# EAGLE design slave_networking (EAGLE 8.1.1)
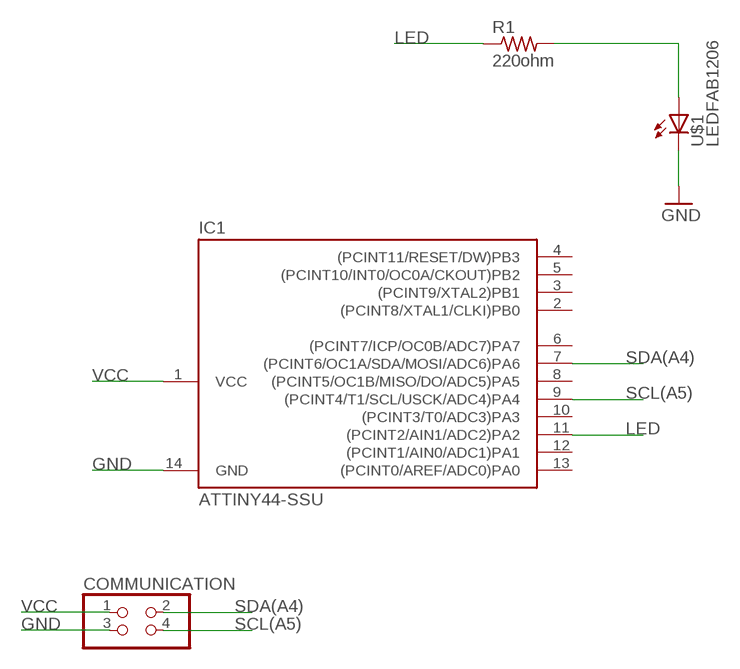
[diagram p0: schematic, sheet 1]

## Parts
COMMUNICATION  PINHD-2X2-SMD  [2X02SMD]
IC1  ATTINY44-SSU  [SOIC14]
R1  220ohm  RES-US1206FAB  [R1206FAB]
U$1  LEDFAB1206  [LED1206FAB]

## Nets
GND: COMMUNICATION.3 IC1.14(GND) U$1.2(C)
LED: IC1.11((PCINT2/AIN1/ADC2)PA2) R1.1
N$1: R1.2 U$1.1(A)
SCL(A5): COMMUNICATION.4 IC1.9((PCINT4/T1/SCL/USCK/ADC4)PA4)
SDA(A4): COMMUNICATION.2 IC1.7((PCINT6/OC1A/SDA/MOSI/ADC6)PA6)
VCC: COMMUNICATION.1 IC1.1(VCC)
Unconnected: IC1.2((PCINT8/XTAL1/CLKI)PB0) IC1.3((PCINT9/XTAL2)PB1) IC1.4((PCINT11/RESET/DW)PB3) IC1.5((PCINT10/INT0/OC0A/CKOUT)PB2) IC1.6((PCINT7/ICP/OC0B/ADC7)PA7) IC1.8((PCINT5/OC1B/MISO/DO/ADC5)PA5) IC1.10((PCINT3/T0/ADC3)PA3) IC1.12((PCINT1/AIN0/ADC1)PA1) IC1.13((PCINT0/AREF/ADC0)PA0)

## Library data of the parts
COMMUNICATION = fab:PINHD-2X2-SMD
IC1 = fab:ATTINY44
R1 = fab:RES-US: Resistor (US Symbol)
U$1 = fab:LED: LED

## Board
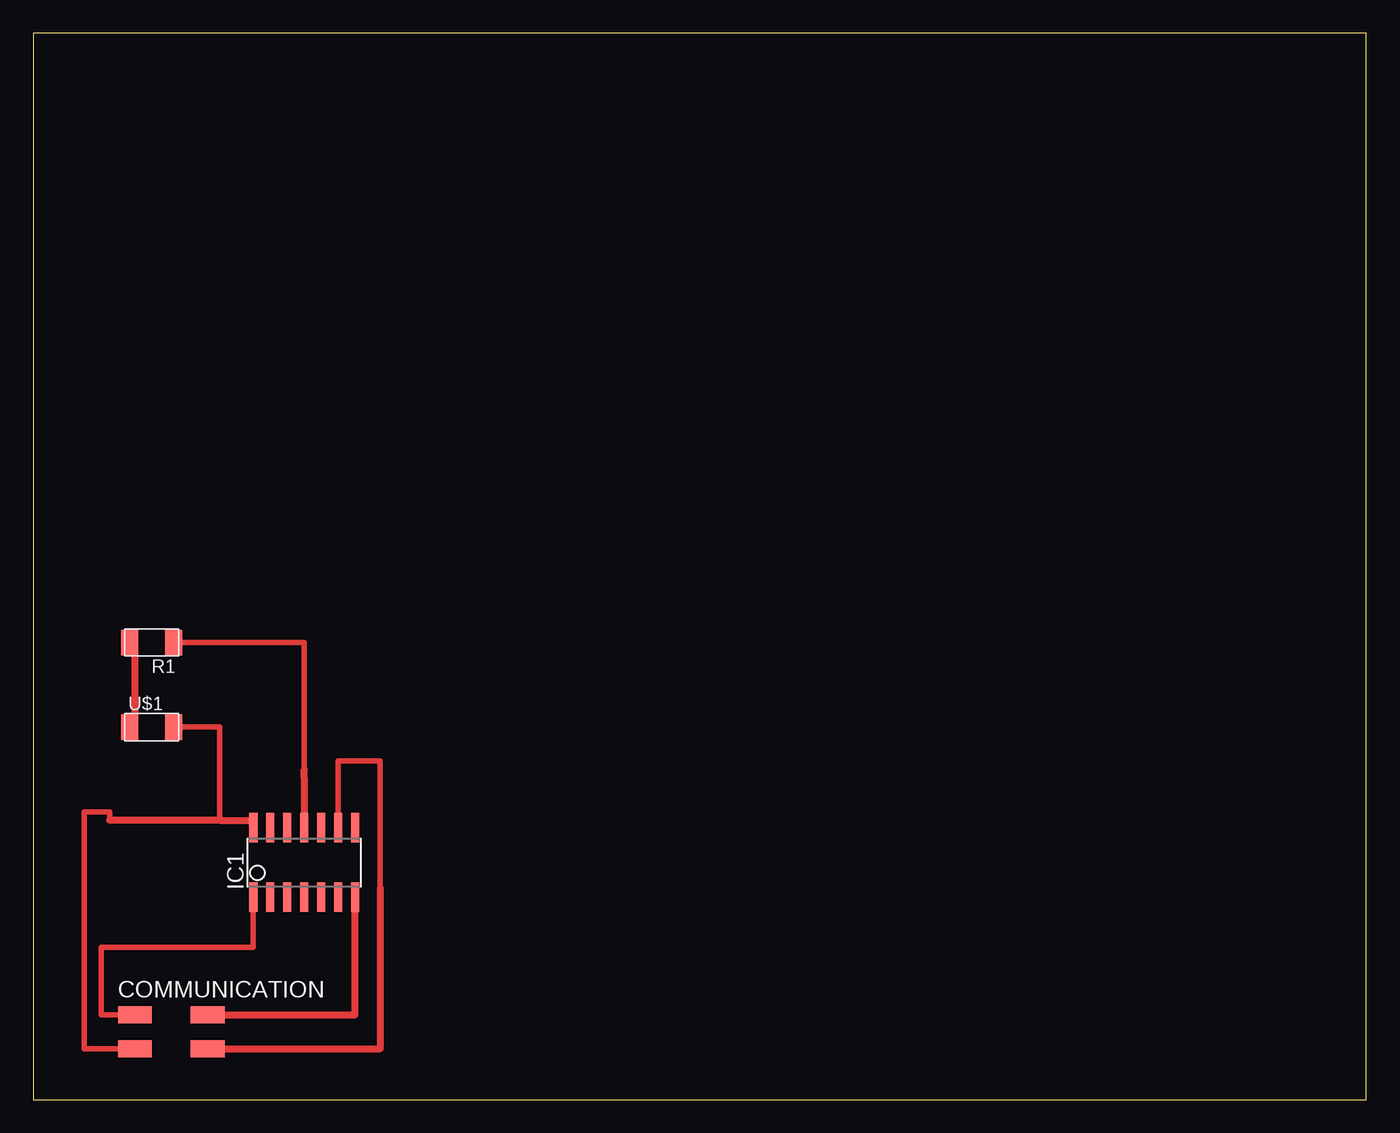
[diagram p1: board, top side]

Size 100 x 80 mm. Coordinates in mm from the lower left corner, seen from the top.
Outline: 0,0 100,0 100,80 0,80 0,0
Copper layers (1*16): Top 0.035mm / dielectric 1.5mm / Bottom 0.035mm
Design rules "default *": minimum track width 20mil, minimum drill 24mil, track to track 32mil, track to pad 8mil, pad to pad 8mil, via to via 8mil, smd to smd 8mil, copper to edge 40mil, drill to drill 8mil, minimum pad ring 10mil, minimum via ring 8mil, stop-mask expansion 4mil, vias tented up to drill 0mil, thermal gap 10mil

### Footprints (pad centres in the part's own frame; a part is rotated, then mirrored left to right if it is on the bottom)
2X02SMD = smd 2.54 x 1.27: 1 -2.54,1.27; 2 2.92,1.27; 3 -2.54,-1.27; 4 2.92,-1.27
SOIC14 = smd 0.61 x 2.21: 1 -3.81,-2.603; 2 -2.54,-2.603; 3 -1.27,-2.603; 4 0,-2.603; 5 1.27,-2.603; 6 2.54,-2.603; 7 3.81,-2.603; 8 3.81,2.603; 9 2.54,2.603; 10 1.27,2.603; 11 0,2.603; 12 -1.27,2.603; 13 -2.54,2.603; 14 -3.81,2.603
R1206FAB = smd 1.27 x 1.905: 1 -1.651,0; 2 1.651,0
LED1206FAB = smd 1.27 x 1.905: 1 -1.651,0; 2 1.651,0

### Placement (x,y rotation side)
COMMUNICATION  10.16,5.08 0 top
IC1  20.32,17.78 0 top
R1  8.89,34.29 180 top
U$1  8.89,27.94 0 top

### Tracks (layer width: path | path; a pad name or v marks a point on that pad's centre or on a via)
GND
  Top 0.406: COMMUNICATION.3 3.81,3.81 3.81,21.59 5.71,21.59 5.71,20.95 | U$1.2 13.97,27.94 13.97,20.95
  Top 0.508: 5.71,20.95 13.97,20.95 16.51,20.95 IC1.14 | 10.79,27.94 U$1.2
LED
  Top 0.406: R1.1 20.32,34.29 20.32,24.13
  Top 0.508: IC1.11 20.32,24.13 20.32,24.77 | 10.79,34.29 R1.1
N$1
  Top 0.508: U$1.1 7.62,27.94 7.62,34.29 R1.2
SCL(A5)
  Top 0.406: IC1.9 22.86,25.4 26.04,25.4 26.04,15.88
  Top 0.508: 26.04,15.88 26.04,3.81 COMMUNICATION.4
SDA(A4)
  Top 0.508: IC1.7 24.13,6.35 COMMUNICATION.2
VCC
  Top 0.406: COMMUNICATION.1 5.08,6.35 5.08,11.43 16.51,11.43 16.51,14.61
  Top 0.508: 8.26,6.35 COMMUNICATION.1 | 16.51,14.61 IC1.1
